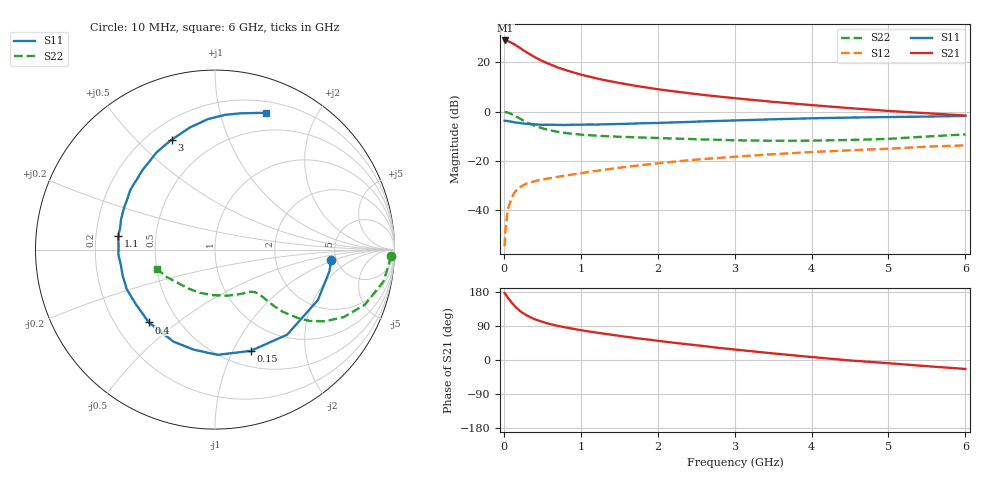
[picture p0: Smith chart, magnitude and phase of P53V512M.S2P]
! SIEMENS Small Signal Semiconductors
! BFP183
! Si NPN RF Bipolar Junction Transistor in SOT143
! VCE = 3.5 V  IC = 12 mA
! Common Emitter S-Parameters:  March  1996
# GHz  S  MA  R  50
!  f  S11  S21  S12  S22
! GHz  MAG  ANG  MAG  ANG  MAG  ANG  MAG  ANG
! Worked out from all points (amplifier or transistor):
!   36 points, 10 MHz to 6 GHz, reference 50 ohm
!   highest |S21| = 29.0 dB at 20 MHz (marker M1)
!   |S21| within 3 dB of that: start of sweep to 207.1 MHz
!   unconditionally stable (mu >= 1): 1.097 GHz to 5.571 GHz
!   at 250 MHz: K = 0.36, MSG = 27.6 dB, |S12| = -30.1 dB
!   at 1.4 GHz: K = 1.09, MAG = 16.0 dB, |S12| = -23.3 dB
!   at 6 GHz: K = 0.94, MSG = 6.1 dB, |S12| = -13.8 dB
!   S11 on the Smith chart (normalised r, x): 10 MHz: 4.52, -0.90; 150 MHz: 0.67, -1.18; 400 MHz: 0.34, -0.40; 1.1 GHz: 0.30, +0.06; 3 GHz: 0.30, +0.64; 6 GHz: 0.31, +1.39
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0.01  0.6496 -5.1  28.07 176.9  0.0018 84.0  0.9822 -2.1
0.02  0.6492 -10.5  28.12 174.2  0.0037 88.2  0.9737 -4.4
0.05  0.6386 -26.1  27.41 165.1  0.0099 80.7  0.9554 -10.7
0.1  0.6215 -49.7  25.18 151.8  0.0172 68.2  0.8895 -20.2
0.15  0.5983 -70.6  22.75 140.3  0.0237 60.9  0.8094 -27.7
0.2  0.5865 -88.6  20.26 131.0  0.0281 54.5  0.7314 -33.1
0.25  0.57 -102.1  17.89 123.4  0.0312 51.4  0.6607 -37.0
0.3  0.5626 -114.3  16 117.5  0.0341 48.2  0.6003 -39.5
0.4  0.5482 -132.2  12.9 107.7  0.0379 45.1  0.5133 -42.5
0.5  0.5357 -145.4  10.68 100.7  0.0411 43.4  0.4553 -43.7
0.6  0.5389 -155.8  9.177 94.9  0.0437 43.3  0.4146 -44.3
0.7  0.5348 -164.1  7.908 90.2  0.0466 43.7  0.3858 -44.6
0.9  0.5388 -176.9  6.303 82.4  0.0524 45.0  0.3508 -45.2
1.1  0.5441 171.9  5.192 75.4  0.0589 45.6  0.3292 -46.5
1.5  0.5577 155.2  3.828 63.7  0.0713 46.4  0.3057 -50.4
1.8  0.577 144.7  3.184 55.7  0.0812 46.1  0.2942 -54.8
2.2  0.5998 132.3  2.593 45.8  0.0946 44.5  0.2816 -62.0
3  0.6577 111.6  1.872 27.7  0.1199 39.6  0.2594 -80.5
3.5  0.6947 101.6  1.575 17.4  0.1349 36.1  0.2539 -94.0
4.5  0.7533 85.6  1.172 -1.2  0.1621 28.0  0.2633 -124.8
5.5  0.7891 74.6  0.924 -16.3  0.1922 21.0  0.3096 -150.5
6  0.8131 69.7  0.829 -23.6  0.2045 16.5  0.3419 -161.8
